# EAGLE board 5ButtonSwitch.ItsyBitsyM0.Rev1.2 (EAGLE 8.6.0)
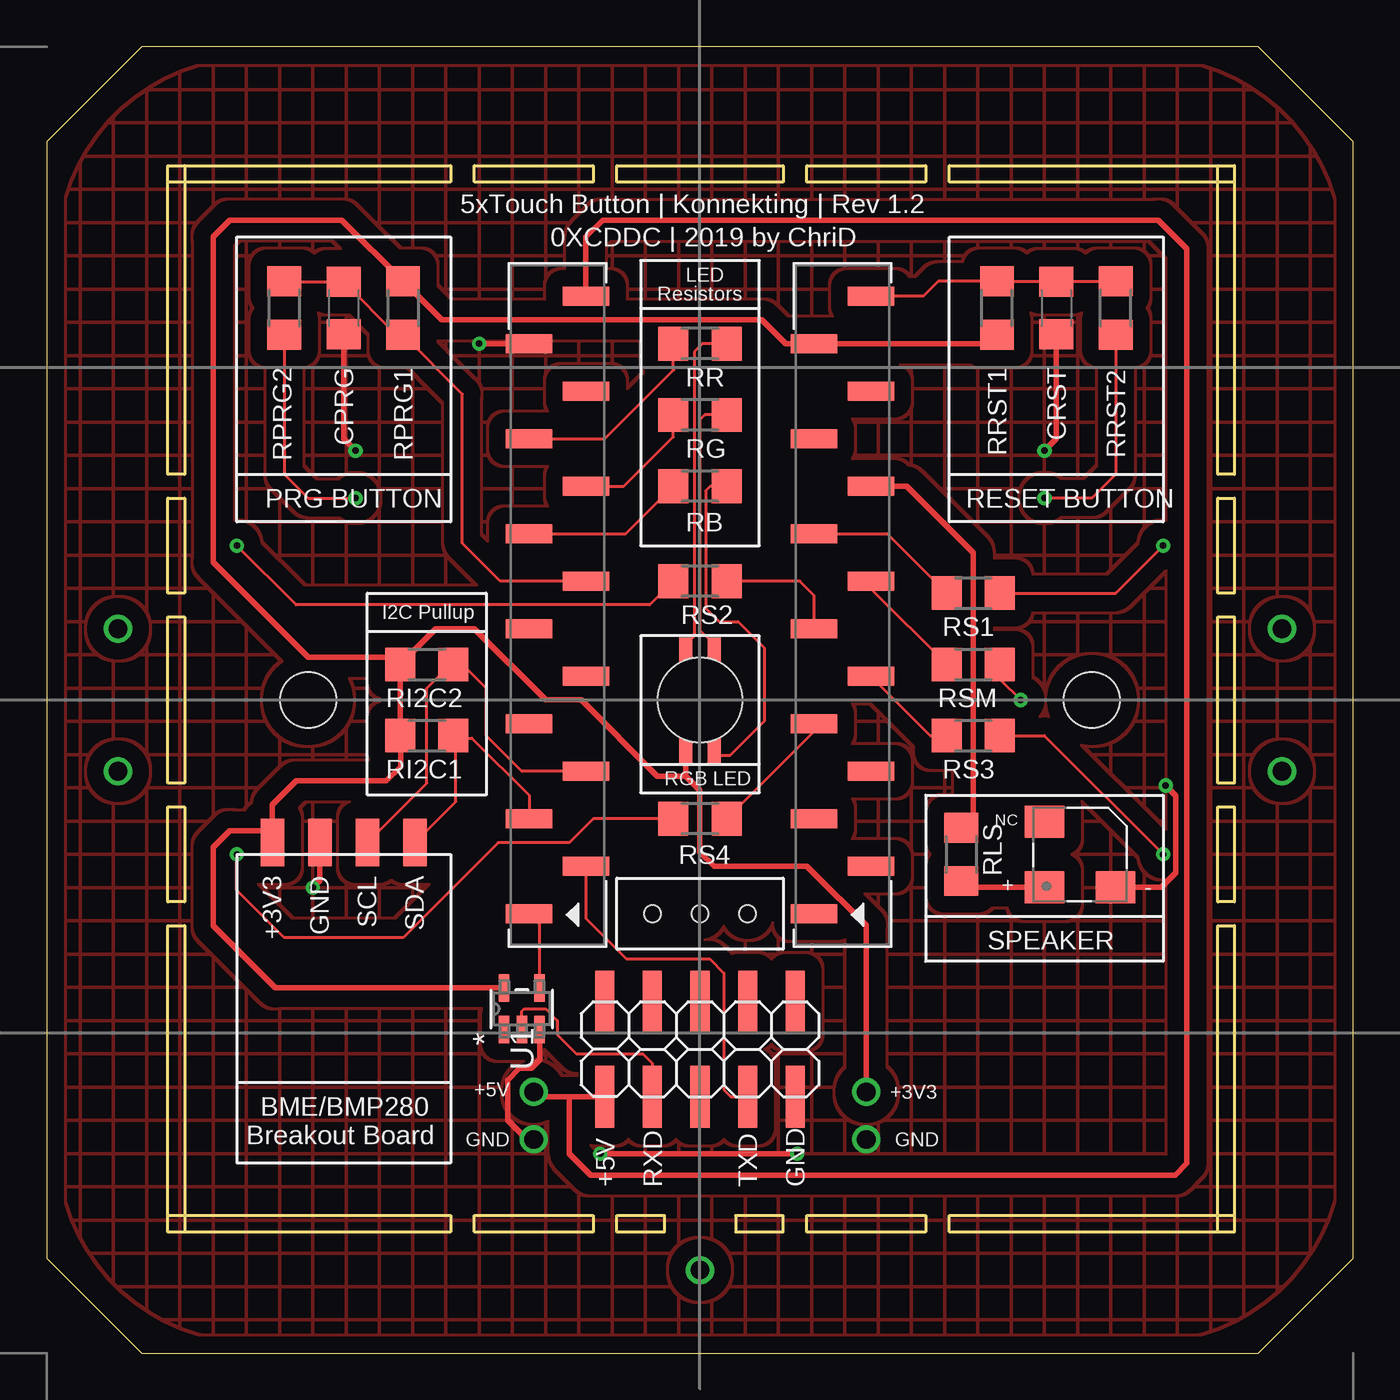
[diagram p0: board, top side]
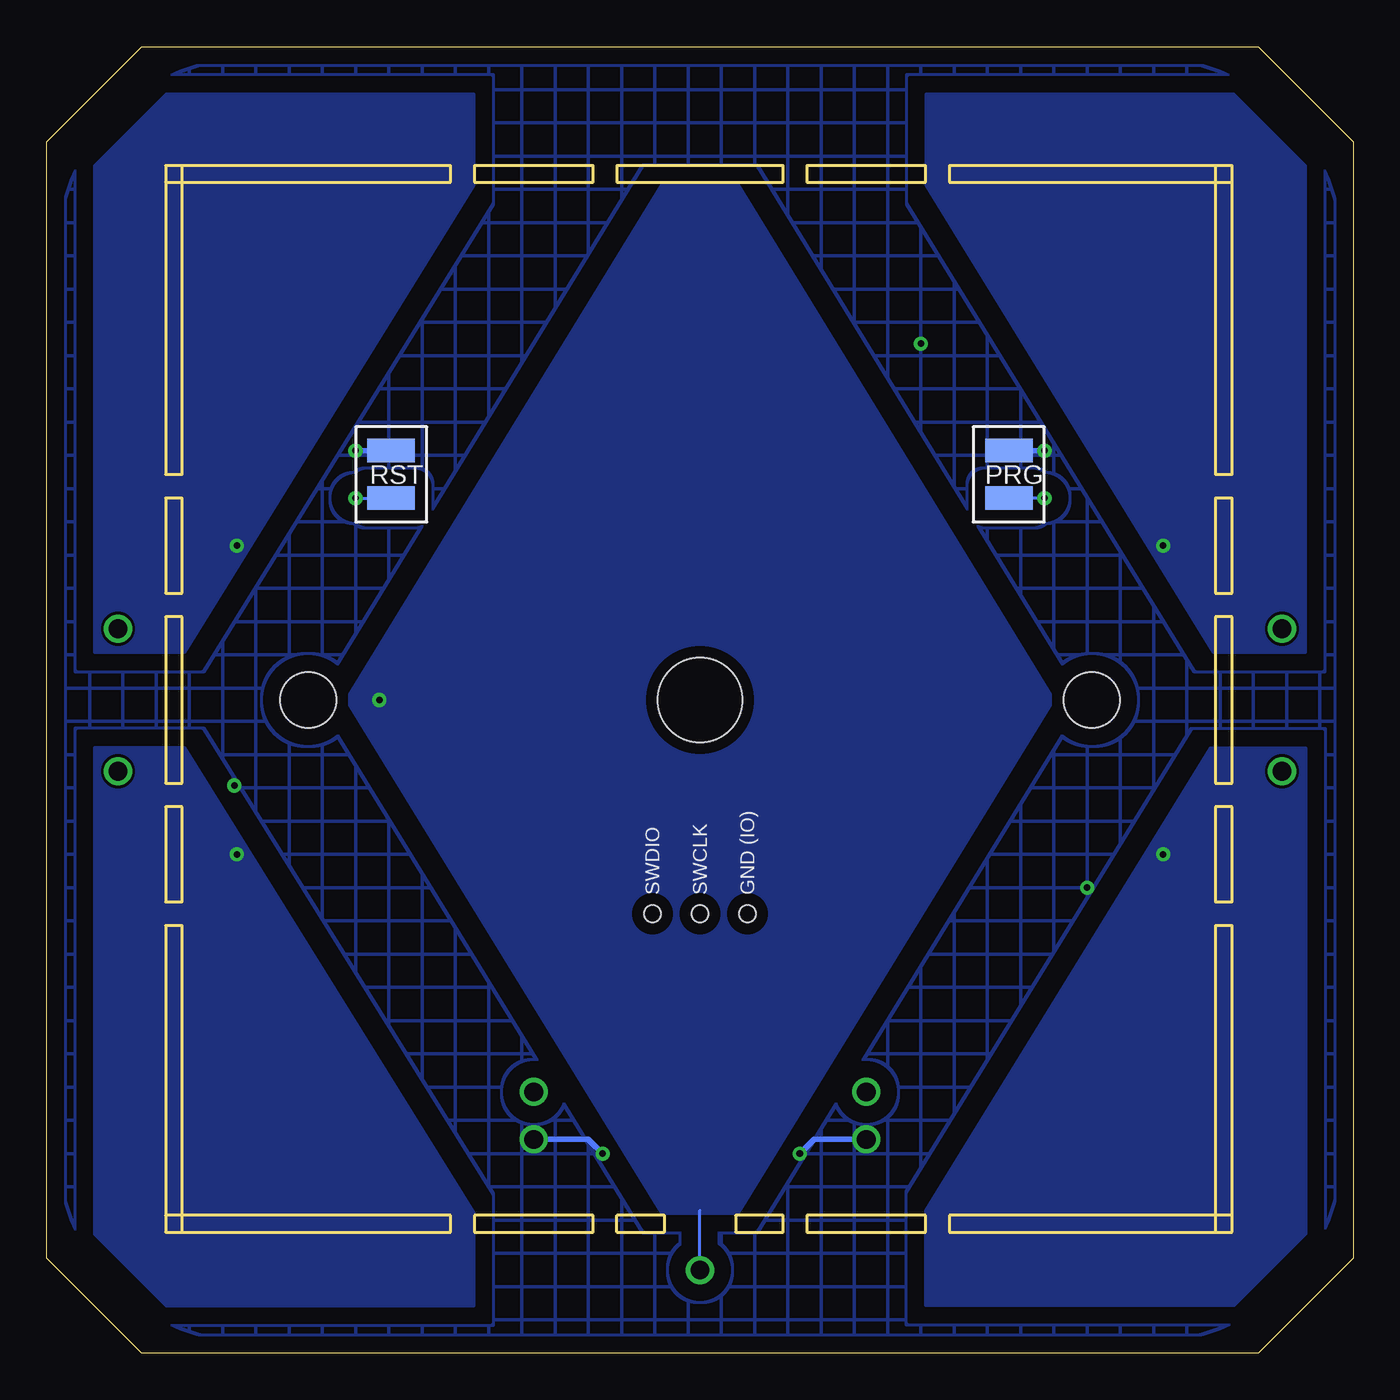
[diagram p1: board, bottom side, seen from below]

Size 69.85 x 69.85 mm. Coordinates in mm from the lower left corner, seen from the top.
Outline: 5.08,69.85 64.77,69.85 69.85,64.77 69.85,5.08 64.77,0 5.08,0 0,5.08 0,64.77 5.08,69.85
Outline: 6.34,69.84 5.08,69.85
Copper layers (1*16): Top 0.035mm / dielectric 1.5mm / Bottom 0.035mm
Design rules "konnektduino": minimum track width 6mil, minimum drill 0.35mm, track to track 6mil, track to pad 6mil, pad to pad 6mil, via to via 6mil, smd to smd 6mil, copper to edge 25mil, drill to drill 6mil, minimum pad ring 10mil, minimum via ring 8mil, stop-mask expansion 1mil, vias tented up to drill 25mil, thermal gap 10mil
Holes 0.9 mm at 37.47,23.5 34.92,23.5 32.38,23.5
Holes 3 mm at 13.97,34.92 55.88,34.92
Milling: 84 lines

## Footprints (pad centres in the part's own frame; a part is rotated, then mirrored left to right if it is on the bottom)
SMD1,27-2,54 = smd 1.27 x 2.54: 1 0,0
C1206 = smd 1.6 x 1.8: 1 -1.4,0; 2 1.4,0
1X14_SMT = smd 1 x 2.5: 1 -16.51,1.52; 2 -13.97,-1.52; 3 -11.43,1.52; 4 -8.89,-1.52; 5 -6.35,1.52; 6 -3.81,-1.52; 7 -1.27,1.52; 8 1.27,-1.52; 9 3.81,1.52; 10 6.35,-1.52; 11 8.89,1.52; 12 11.43,-1.52; 13 13.97,1.52; 14 16.51,-1.52
CUI_CSS-0575B-SMT = smd 2.1 x 1.7: 1 -1.9,-1.75; 2 1.9,-1.75; 3 -1.9,1.75
R1206 = smd 1.6 x 1.803: 1 -1.422,0; 2 1.422,0
2X05SMD = smd 1.016 x 3.302: 1 -1.27,-3.81; 2 -1.27,1.27; 3 1.27,-3.81; 4 1.27,1.27; 5 3.81,-3.81; 6 3.81,1.27; 7 6.35,-3.81; 8 6.35,1.27; 9 8.89,-3.81; 10 8.89,1.27
DBV5 = smd 1.473 x 0.559: 1 -1.118,0.95; 2 -1.118,0; 3 -1.118,-0.95; 4 1.118,-0.95; 5 1.118,0.95
PLCC4R_EX = smd 1.4 x 0.7: 1 -2.667,-0.762; 2 2.64,-0.762; 3 2.64,0.762; 4 -2.667,0.762 | hole 4.5: 0,0

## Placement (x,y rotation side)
+3V3  WIREPADSMD1,27-254  [SMD1,27-2,54]  12.06,27.3 0 top
CPRG  100nF  [C1206]  15.88,55.88 270 top
CRST  100nF  [C1206]  53.98,55.88 270 top
GND  WIREPADSMD1,27-254  [SMD1,27-2,54]  14.61,27.3 0 top
ITSYBITSYM0  [1X14_SMT]  42.55,40.01 90 top
JP1  [1X14_SMT]  27.3,40.01 90 top
LS1  CSS-0575B-SMT  [CUI_CSS-0575B-SMT]  55.24,26.67 0 top
PAD_GND1  WIREPADSMD1,27-254  [SMD1,27-2,54]  18.41,48.26 90 bottom
PAD_GND2  WIREPADSMD1,27-254  [SMD1,27-2,54]  51.44,48.26 90 bottom
PAD_PRG  WIREPADSMD1,27-254  [SMD1,27-2,54]  18.41,45.72 90 bottom
PAD_RST  WIREPADSMD1,27-254  [SMD1,27-2,54]  51.44,45.72 90 bottom
RB  330  [R1206]  34.92,46.35 0 top
RG  330  [R1206]  34.92,50.16 0 top
RI2C1  10k  [R1206]  20.32,33.02 180 top
RI2C2  10k  [R1206]  20.32,36.83 180 top
RLS  0  [R1206]  48.9,26.67 90 top
RPRG1  10k  [R1206]  19.05,55.88 90 top
RPRG2  330E  [R1206]  12.7,55.88 270 top
RR  330  [R1206]  34.92,53.98 0 top
RRST1  10k  [R1206]  50.8,55.88 270 top
RRST2  330E  [R1206]  57.15,55.88 270 top
RS1  1k  [R1206]  49.53,40.64 180 top
RS2  1k  [R1206]  34.92,41.27 0 top
RS3  1k  [R1206]  49.53,33.02 180 top
RS4  1k  [R1206]  34.92,28.57 0 top
RSM  1k  [R1206]  49.53,36.83 180 top
SAM12235-ND  SIEMENS BCU  [2X05SMD]  31.11,17.53 0 top
SCL  WIREPADSMD1,27-254  [SMD1,27-2,54]  17.14,27.3 0 top
SDA  WIREPADSMD1,27-254  [SMD1,27-2,54]  19.68,27.3 0 top
U1  SN74LV1T34DBVR  [DBV5]  25.4,18.41 90 top
U$4  QBLP677R-RGB-EX  [PLCC4R_EX]  34.92,34.92 90 top

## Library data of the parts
+3V3 GND PAD_GND1 PAD_GND2 PAD_PRG PAD_RST SCL SDA = wirepad
CPRG CRST = rcl; SPICEPREFIX: C
ITSYBITSYM0 JP1 = pinhead+
LS1 = CSS-0575B-SMT; CUI_PURCHASE_URL: https://www.cui.com/product/audio/buzzers/audio-transducers/css-0575b-smt?utm_source=snapeda.com&utm_medium=referral&utm_campaign=snapedaBOM; DESCRIPTION: AUDIO MAGNETIC XDCR 2-4V SMD; DIGI-KEY_PART_NUMBER: 102-2202-1-ND; DIGI-KEY_PURCHASE_URL: https://www.digikey.com/product-detail/en/cui-inc/CSS-0575B-SMT-TR/102-2202-1-ND/2364651?utm_source=snapeda&utm_medium=aggregator&utm_campaign=symbol; MF: CUI Inc.; MP: CSS-0575B-SMT-TR; PACKAGE: CUI Inc.
RB RG RI2C1 RI2C2 RLS RPRG1 RPRG2 RR RRST1 RRST2 RS1-RS4 RSM = resistor
SAM12235-ND = pinhead
U1 = SN74LV1T34DBVR; MANUFACTURER_PART_NUMBER: SN74LV1T34DBVR; VENDOR: Texas Instruments
U$4 = ChriD_TouchSwitch

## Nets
+3V3: +3V3.1 ITSYBITSYM0.13 RI2C1.2 RI2C2.2 RPRG1.2 RRST1.2 U1.5 U$4.4
+5V: JP1.14 SAM12235-ND.1
A0: ITSYBITSYM0.10 RLS.2
A1: ITSYBITSYM0.9 RS1.2
A2: ITSYBITSYM0.8 RSM.2
A3: ITSYBITSYM0.7 RS2.2
A4: ITSYBITSYM0.6 RS3.2
A5: ITSYBITSYM0.5 RS4.2
D7: JP1.6
D9: JP1.7
D10: CPRG.1 JP1.8 RPRG1.1 RPRG2.1
D11: JP1.9 RB.1
D12: JP1.10 RG.1
D13: JP1.11 RR.1
GND: CPRG.2 CRST.2 GND.1 JP1.13 LS1.2 PAD_GND1.1 PAD_GND2.1 SAM12235-ND.9 U1.3
LS_USART1_RX: SAM12235-ND.3 U1.2
MISO: ITSYBITSYM0.2
MOSI: ITSYBITSYM0.3
N$1: RB.2 U$4.1
N$2: RG.2 U$4.2
N$3: RR.2 U$4.3
N$4: LS1.1 RLS.1
PRG: PAD_PRG.1 RPRG2.2
RESET: PAD_RST.1 RRST2.2
RST: CRST.1 ITSYBITSYM0.14 RRST1.1 RRST2.1
SCK: ITSYBITSYM0.4
SCL: JP1.4 RI2C2.1 SCL.1
SDA: JP1.3 RI2C1.1 SDA.1
SENSPAD_1: RS1.1
SENSPAD_2: RS2.1
SENSPAD_3: RS3.1
SENSPAD_4: RS4.1
SENSPAD_MAIN: RSM.1
USART1_RX: JP1.1 U1.4
USART1_TX: JP1.2 SAM12235-ND.7

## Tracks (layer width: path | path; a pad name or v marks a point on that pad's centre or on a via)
+3V3  (via drill 1)
  Top 0.152: U$4.4 34.16,31.89
  Top 0.305: RRST1.2 50.32,53.98 ITSYBITSYM0.13 39.5,53.98 38.23,55.24 21.11,55.24 RPRG1.2 15.77,60.58 9.78,60.58 8.89,59.69 8.89,42.29 13.97,37.21 14.92,37.21 18.26,37.21 18.9,36.58 | 18.9,36.58 RI2C2.2 20.8,38.73 22.86,38.73 26.67,34.92 28.57,34.92 32.64,30.86 34.16,30.86 | 18.9,36.58 RI2C1.2 18.92,32.99 18.92,31.37 18.16,30.61 13.34,30.61 12.06,29.34 12.06,27.94 | +3V3.1 12.06,27.94 | v43.81,13.97 43.81,22.89 42.4,24.3 42.38,24.3 40.64,26.04 35.69,26.04 34.92,26.8 34.92,30.1 34.16,30.86 | 34.16,31.89 34.16,30.86 | U1.5 12.22,19.53 8.89,22.86 8.89,27.05 9.78,27.94 12.06,27.94
+5V  (via drill 1)
  Top 0.305: JP1.14 28.82,59.69 29.72,60.58 59.44,60.58 60.96,59.05 60.96,10.16 60.33,9.53 29.08,9.53 27.94,10.67 27.94,13.72 | 29.59,13.97 SAM12235-ND.1 27.94,13.72 | 27.94,13.72 26.29,13.72 v26.04,13.97
A0
  Top 0.305: ITSYBITSYM0.10 45.97,46.35 49.53,42.8 49.53,28.73 RLS.2
A1
  Top 0.152: ITSYBITSYM0.9 44.93,43.81 RS1.2
A2
  Top 0.152: ITSYBITSYM0.8 44.06,40.87 RSM.2
A3
  Top 0.152: ITSYBITSYM0.7 41.02,40.51 40.26,41.27 RS2.2
A4
  Top 0.152: ITSYBITSYM0.6 47.24,33.02 RS3.2
A5
  Top 0.152: RS4.2 41.02,33.25 ITSYBITSYM0.5
D10
  Top 0.152: RPRG2.1 12.72,57.28 CPRG.1 18.7,54.46 RPRG1.1 22.23,51.28 22.23,43.31 24.26,41.27 JP1.8
D11
  Top 0.152: JP1.9 30.96,43.81 RB.1
D12
  Top 0.152: 29.69,46.35 JP1.10 30.86,46.35 33.5,49 RG.1
D13
  Top 0.152: JP1.11 29.84,48.9 33.53,52.58 33.5,52.6 RR.1
GND  (via drill 0.35, 1)
  Top 0.305: GND.1 14.61,25.27 v14.22,24.89 | CPRG.2 15.88,48.9 v16.51,48.26 | CRST.2 53.98,48.9 v53.34,48.26 | JP1.13 v23.11,53.98 | v29.59,10.67 v40.13,10.67 | LS1.2 59.59,24.92 60.37,25.7 60.37,29.8 v59.82,30.35 | U1.3 26.35,15.68 25.91,15.24 25.27,15.24 24.64,14.61 24.64,12.45 25.65,11.43 v26.04,11.43
  Bottom 0.305: v16.51,48.26 PAD_GND1.1 | v53.34,48.26 PAD_GND2.1 | v26.04,11.43 28.83,11.43 v29.59,10.67 | v40.13,10.67 40.89,11.43 v43.81,11.43
  pour Top (isolate 0.889, rank 6, no thermals, hatched): 0.64,10.79 arc90 10.79,0.64 59.05,0.64 arc90 69.22,10.79 69.22,59.05 arc90 59.05,69.22 10.79,69.22 arc90 0.64,59.05
  pour Bottom (isolate 0.889, rank 6, no thermals, hatched): 0.64,10.79 arc90 10.79,0.64 59.05,0.64 arc90 69.22,10.79 69.22,59.05 arc90 59.05,69.22 10.79,69.22 arc90 0.64,59.05
LS_USART1_RX
  Top 0.152: 25.4,17.78 U1.2 25.4,18.29 25.53,18.41 26.67,18.41 27.3,17.78 27.3,17.02 28.32,16 31.88,16 32.38,15.49 SAM12235-ND.3
N$1
  Top 0.152: RB.2 35.48,46.35 35.23,46.1 35.23,39.83 35.94,39.12 36.96,39.12 38.35,37.72 38.35,33.78 36.54,31.96 35.69,31.96 U$4.1
N$2
  Top 0.152: RG.2 35.18,50.16 34.92,49.91 34.92,38.65 35.52,38.06 35.69,37.89 U$4.2
N$3
  Top 0.152: RR.2 35.05,53.98 34.62,53.54 34.62,38.34 34.33,38.06 34.16,37.89 U$4.3
N$4
  Top 0.305: LS1.1 49.22,24.92 RLS.1
PRG  (via drill 0.35)
  Top 0.152: RPRG2.2 12.7,46.99 13.97,45.72 v16.51,45.72
  Bottom 0.152: v16.51,45.72 PAD_PRG.1
RESET  (via drill 0.35)
  Top 0.152: RRST2.2 57.15,46.99 55.88,45.72 v53.34,45.72
  Bottom 0.152: v53.34,45.72 PAD_RST.1
RST
  Top 0.152: RRST2.1 57.13,57.28 CRST.1 50.82,57.28 RRST1.1 47.65,57.3 46.86,56.52 ITSYBITSYM0.14
SCL
  Top 0.152: JP1.4 25.4,31.11 23.5,33.02 23.5,35.56 22.23,36.83 RI2C2.1 21.59,36.83 20.32,35.56 20.32,30.48 SCL.1
SDA
  Top 0.152: RI2C1.1 21.87,32.89 | 21.87,32.89 22.73,32.89 25.79,29.84 JP1.3 | SDA.1 21.87,29.49 21.87,32.89
SENSPAD1  (via drill 1)
  other vias: 66.04,38.73
SENSPAD2  (via drill 1)
  other vias: 3.81,38.73
SENSPAD3  (via drill 1)
  other vias: 66.04,31.11
SENSPAD4  (via drill 1)
  other vias: 3.81,31.11
SENSPAD_1  (via drill 0.35)
  Top 0.152: RS1.1 57.15,40.64 v59.69,43.18
  pour Bottom: 46.99,62.48 46.99,67.31 63.5,67.31 67.31,63.5 67.31,37.47 62.48,37.47
SENSPAD_2  (via drill 0.35)
  Top 0.152: RS2.1 32.23,40.01 13.34,40.01 v10.16,43.18
  pour Bottom: 22.86,62.48 7.49,37.48 2.54,37.47 2.54,63.5 6.35,67.31 22.86,67.31 22.86,64.77
SENSPAD_3  (via drill 0.35)
  Top 0.152: RS3.1 53.34,33.02 v59.69,26.67
  pour Bottom: 46.99,7.49 62.48,32.38 67.31,32.38 67.31,6.35 63.5,2.54 46.99,2.54
SENSPAD_4  (via drill 0.35)
  Top 0.152: RS4.1 29.21,28.57 27.94,27.3 24.13,27.3 19.05,22.23 12.7,22.23 10.16,24.77 v10.16,26.67
  pour Bottom: 22.86,7.62 7.62,32.38 2.54,32.38 2.54,6.35 6.35,2.54 22.86,2.54
SENSPAD_MAIN  (via drill 0.35, 1)
  Top 0.152: RSM.1 50.95,36.04 v52.07,34.92
  Bottom 0.152: v34.92,4.45 34.92,7.62
  pour Bottom: 36.96,62.48 53.85,34.92 36.96,7.49 32.89,7.49 16,34.92 32.89,62.48
USART1_RX
  Top 0.152: U1.4 26.35,22.93 JP1.1
USART1_TX
  Top 0.152: JP1.2 28.82,23.25 30.99,21.08 35.43,21.08 36.2,20.32 36.2,20.07 36.2,14.1 36.58,13.72 SAM12235-ND.7

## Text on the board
tPlace: SPEAKER | BME/BMP280 | Breakout Board
tNames: 5xTouch Button | Konnekting | Rev 1.2 | 0XCDDC | 2019 by ChriD | LED | Resistors | PRG BUTTON | RESET BUTTON | I2C Pullup | RGB LED | +5V | +3V3 | GND | GND | +5V | RXD | TXD | GND
bNames: PRG | RST | GND (IO) | SWCLK | SWDIO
